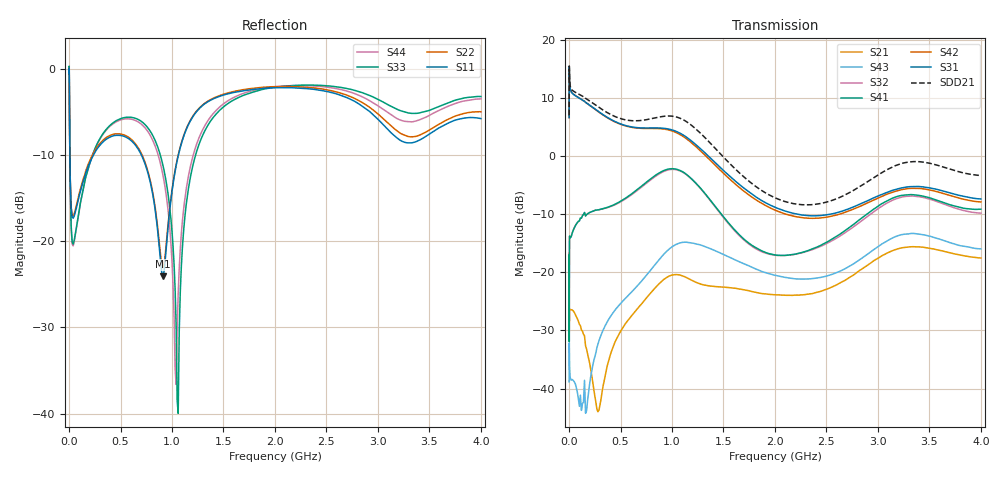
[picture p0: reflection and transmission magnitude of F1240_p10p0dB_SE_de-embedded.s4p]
! Integrated Device Technology
! Corporate Headquarters
! 6024 Silver Creek Valley Road
! San Jose, CA 95138  USA
! Phone:  1-408-284-8200
! Toll Free:  1-800-223-1366
! Webpage:  http://www.idt.com/
! Timing and RF Division
! 515 Groton Road, Suite 102
! Westford, MA 01886-6024
! Device:  F1240
! Description: Dual Intermediate Frequency Digital Variable Gain Amplifier
! Frequency:  10.0 -  500.00 MHz
! Package:  5x5 mm QFN Plastic Package: 32 pin
! Ports:  8 RF, 20 DC
!  Pin  1  = GA3 / Data  Pin 17  = RF OUT_B+
!  Pin  2  = GA4 / CLK  Pin 18  = RF OUT_B-
!  Pin  3  = GA5  Pin 19  = STBY_B
!  Pin  4  = VMODE  Pin 20  = Ground
!  Pin  5  = No Connect  Pin 21  = Ground
!  Pin  6  = GB5  Pin 22  = STB_A
!  Pin  7  = GB4  Pin 23  = RF OUT_A-  = Port 4
!  Pin  8  = GB3  Pin 24  = RF OUT_A+  = Port 3
!  Pin  9  = GB2  Pin 25  = GA0
!  Pin 10  = GB1  Pin 26  = ISET_A
!  Pin 11  = RF IN_B+  Pin 27  = VCC
!  Pin 12  = RF IN_B-  Pin 28  = Ground
!  Pin 13  = Ground  Pin 29  = RF IN_A-  = Port 2
!  Pin 14  = VCC  Pin 30  = RF IN_A+  = Port 1
!  Pin 15  = ISET_B  Pin 31  = GA1
!  Pin 16  = GB0  Pin 32  = GA2 / CSb
! Gain  = +19.5 dB
! State  = 1
! Voltage  = +5.00 V
! Current  = 85.292 mA (one channel only)
! Temperture  =  +25 C
! Test Date  =  2017-10-18
! Board  =  EB4031
! Data:  The device was measured on a custom evaluation board which has
!  individual transmission lines to the RF pins.  Data was collected
!  using a calibrated network analyzer.  The evaluation board was
!  de-embedded using Automatic Fixture Removal.
!  The reference plane is the edge of the package pin.
!  Only Channel A was measured.
!  This data is in single-ended operation.  If your needs are balanced
!  or differential S-parameters then this file needs to be used a
!  linear simulator.
! File Date:  2017-11-10  MJV
! Note:
!  Integrated Device Technology supplies this data as a sample of measured
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# Hz S dB R 100
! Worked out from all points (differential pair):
!   410 points, 500 kHz to 4 GHz, reference 100 ohm
!   strongest paths, dB at 500 kHz, 930 MHz, 1.96 GHz, 2.98 GHz, 4 GHz:
!     S31: 6.6, 4.7, -8.5, -7.0, -7.4
!     S42: 6.6, 4.6, -9.0, -7.4, -7.9
!     S41: -19.6, -2.4, -16.9, -8.9, -9.1
!     S32: -19.4, -2.6, -16.9, -9.3, -9.8
!     S43: -38.8, -16.7, -20.3, -15.9, -16.0
!     S21: -25.9, -21.1, -23.8, -17.8, -17.5
!   taken as a pair (ports 1,2 in; 3,4 out), SDD21 dB: 7.0, 6.8, -6.8, -3.5, -3.3
!   lowest |S11| = -24.0 dB at 910 MHz (marker M1), VSWR 1.13, Z = 110 + j8.07 ohm
!   |S11| at or under -10 dB: 7.87 MHz to 235.1 MHz (227.2 MHz wide, 187 % of centre); 704.4 MHz to 1.061 GHz (356.8 MHz wide, 40.4 % of centre)
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500000  -0.40 -5.7  -25.85 -4.1  -27.23 81.1  -58.65 70.2
        -25.87 -4.0  -0.40 -5.6  -58.40 71.2  -27.22 82.3
        6.61 -105.1  -19.42 61.7  -0.49 1.4  -38.83 -110.3
        -19.57 62.6  6.59 -103.9  -38.84 -109.7  -0.50 3.7
3000000  -3.09 -58.9  -28.34 -8.7  -16.38 23.1  -50.59 56.7
         -28.31 -8.6  -3.06 -58.9  -50.46 56.2  -16.38 23.3
         14.68 -178.2  -17.80 9.6  -2.60 -54.5  -33.53 113.2
         -17.55 9.3  14.68 -178.0  -33.53 113.6  -2.66 -54.2
2e8  -10.87 -132.0  -35.52 -73.2  -18.52 -50.6  -34.23 16.6
     -35.64 -70.3  -10.62 -133.0  -34.22 17.2  -18.54 -50.7
     8.74 109.6  -9.72 -26.0  -10.96 -95.1  -39.57 137.6
     -9.72 -26.4  8.72 108.9  -39.17 127.0  -11.00 -94.1
5.3e8  -7.76 179.4  -29.94 -10.4  -19.78 -108.3  -28.53 -56.4
       -29.31 -12.7  -7.60 178.3  -28.66 -54.4  -19.90 -108.6
       5.34 26.7  -7.58 -89.2  -5.62 -157.0  -25.81 15.0
       -7.46 -90.7  5.27 25.8  -24.80 12.2  -5.78 -156.9
9.1e8  -24.04 35.4  -21.46 -83.2  -17.61 170.3  -25.05 -145.9
       -21.39 -90.4  -23.05 35.0  -25.32 -139.7  -17.92 169.7
       4.78 -67.7  -2.74 173.0  -11.04 138.0  -18.02 -66.4
       -2.58 169.0  4.66 -69.4  -17.09 -71.2  -12.16 139.4
1.22e9  -5.19 -113.8  -20.61 -168.8  -19.62 85.2  -25.22 139.1
        -21.62 -172.0  -5.12 -113.6  -24.92 146.3  -20.25 84.2
        2.13 -159.7  -4.50 64.1  -10.34 -100.4  -15.61 -160.7
        -4.45 59.3  1.80 -161.6  -15.05 -165.2  -9.38 -105.1
4e9  -5.71 -152.1  -17.65 76.2  -20.74 -60.6  -20.78 -47.9
     -17.55 75.6  -4.92 -148.5  -22.35 -28.6  -22.95 -53.2
     -7.39 19.3  -9.83 -100.8  -3.15 -138.8  -16.53 86.7
     -9.14 -114.1  -7.91 27.6  -15.97 60.8  -3.42 -145.5
